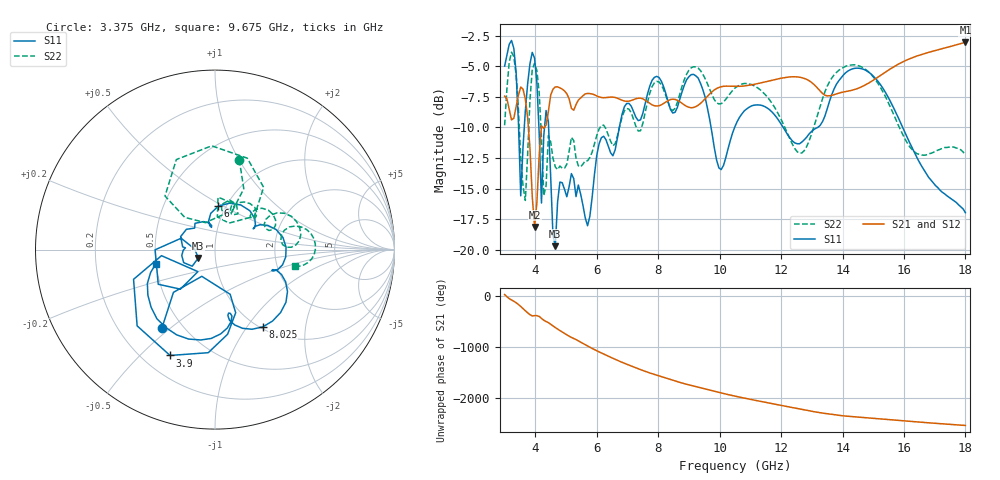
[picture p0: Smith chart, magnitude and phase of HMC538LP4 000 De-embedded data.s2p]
! Chelmsford, MA 01824
! http://www.hittite.com
! Tel: 978-250-3343
! Fax: 978-250-3373
! Device  :  HMC538LP4
! Description:  600 Analog Phase Shifter
! Frequency  :  6.0 GHz - 15.0 GHz
! Package  :  LP4  - 4x4 mm Quad Flatpack No-Lead (QFN) Plastic Package: 24 pin
! Ports  :  2 RF, 1 DC
!  Pin  3  = Rfin  = Port 1
!  Pin  16  = Rfout = Port 2
!  pin  21  = vCTL
! Voltages:  VCTL  = 0 to 5.0 Volts
! Currents :  Vb(V)  Vd(V)  Ib(mA)  Id(mA)
!  0.00  0.00  0.000000  0.485550
! Data:  The device was measured on evaluation board 111296-1.
!  Data was collected using a calibrated network analyzer.
!  The evaluation circuit board was modeled and simulated.This was use
!  to removed the evaluation board circuit from the measured data.
!  The reference plane is the center of the package pin.
! Misc:  Lot #
!Date Measured:  03 - 11 -2009
! Date:  03 - 17 -2009
! Note:
!  Hittite Microwave supplies this data as a sample of measured data at the
!  package pin for this package product.  Your particular data for this product
!  may vary.
!  Data was taken at 25 degrees C.
!  Hittite Microwave reserves the right to change this data at anytime.
# MHz S MA R 50
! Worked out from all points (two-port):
!   201 points, 3 GHz to 18 GHz, reference 50 ohm
!   highest |S21| = -3.04 dB at 18 GHz (marker M1); lowest = -18.1 dB at 3.975 GHz (marker M2)
!   |S21| within 3 dB of the highest: 11.9 GHz to 12.79 GHz (896.7 MHz wide, 7.26 % of centre); 15.07 GHz to end of sweep
!   lowest |S11| = -19.7 dB at 4.65 GHz (marker M3), VSWR 1.23, Z = 41.4 - j3.84 ohm
!   |S11| at or under -10 dB: 4.433 GHz to 6.736 GHz (2.303 GHz wide, 41.2 % of centre); 12.07 GHz to 13.19 GHz (1.124 GHz wide, 8.9 % of centre); 15.96 GHz to end of sweep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
!   |S22| runs from -16.0 to -3.9 dB; largest |S21 - S12| = 0.0021
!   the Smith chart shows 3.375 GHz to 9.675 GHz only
!   S11 on the Smith chart (normalised r, x): 3.375 GHz: 0.38, -0.47; 3.9 GHz: 0.31, -0.62; 6 GHz: 0.92, +0.47; 8.025 GHz: 1.03, -1.19; 9.675 GHz: 0.50, -0.09
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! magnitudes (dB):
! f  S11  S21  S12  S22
! 3 GHz  -5.0  -7.4  -7.4  -9.8
! 3.15 GHz  -3.2  -8.5  -8.5  -4.7
! 3.375 GHz  -5.5  -8.3  -8.3  -5.7
! 3.525 GHz  -15.6  -6.7  -6.7  -12.5
! 3.675 GHz  -8.6  -7.7  -7.7  -16.0
! 3.9 GHz  -3.9  -15.6  -15.6  -5.3
! 3.975 GHz  -4.3  -18.1  -18.1  -4.8
! 4.2 GHz  -16.2  -9.9  -9.9  -10.8
! 4.275 GHz  -10.7  -10.1  -10.1  -15.6
! 4.425 GHz  -9.5  -8.7  -8.7  -10.7
! 4.65 GHz  -19.7  -6.7  -6.7  -13.2
! 4.8 GHz  -14.5  -6.8  -6.8  -13.2
! 5.55 GHz  -16.4  -7.4  -7.4  -13.0
! 6 GHz  -12.3  -7.4  -7.4  -10.7
! 8.025 GHz  -5.9  -8.2  -8.2  -6.3
! 9.675 GHz  -9.3  -7.3  -7.3  -6.9
! 10.05 GHz  -13.4  -6.7  -6.7  -8.1
! 10.5 GHz  -9.9  -6.6  -6.7  -6.8
! 13.05 GHz  -10.2  -6.4  -6.5  -10.1
! 14.1 GHz  -5.5  -7.1  -7.1  -5.0
! 15.53 GHz  -7.7  -5.3  -5.3  -8.2
! 18 GHz  -17.0  -3.0  -3.0  -12.2
